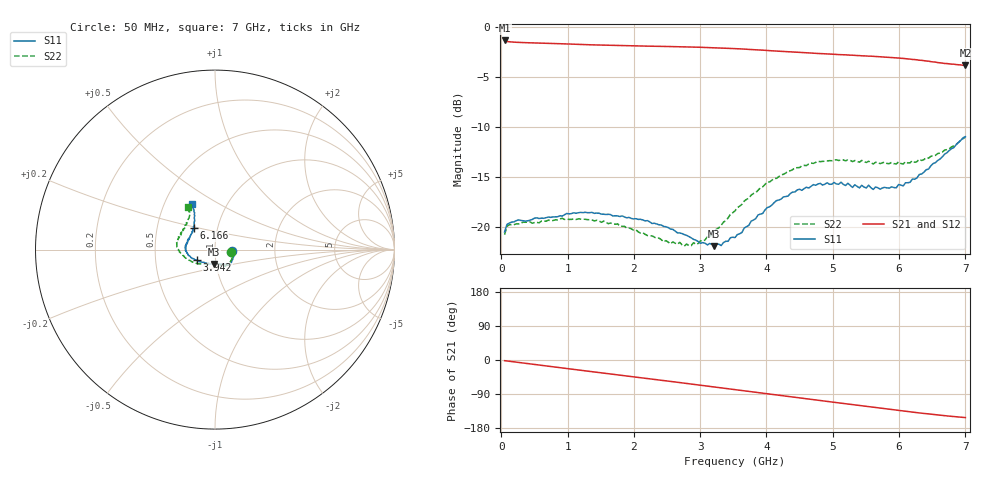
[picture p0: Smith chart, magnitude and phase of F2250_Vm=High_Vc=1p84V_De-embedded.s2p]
! Integrated Device Technology
! Corporate Headquarters
! 6024 Silver Creek Valley Road
! San Jose, CA 95138  USA
! Phone:  1-408-284-8200
! Toll Free:  1-800-223-1366
! Webpage:  http://www.idt.com/
! Timing and RF Division
! 515 Groton Road, Suite 102
! Westford, MA 01886-6024
! Device:  F2250
! Description: Voltage Variable RF Attenuator
! Frequency:  50.0 -  6000.00 MHz
! Package:  3x3 mm Thin QFN Plastic Package: 16 pin
! Ports:  2 RF, 3 DC
!  Pin  1  = GND
!  Pin  2  = NC
!  Pin  3  = RF1  = Port 1
!  Pin  4  = NC
!  Pin  5  = GND
!  Pin  6  = GND
!  Pin  7  = GND
!  Pin  8  = GND
!  Pin  9  = NC
!  Pin 10  = RF2  = Port 2
!  Pin 11  = NC
!  Pin 12  = GND
!  Pin 13  = GND
!  Pin 14  = VCNTRL
!  Pin 15  = VDD
!  Pin 16  = VMODE
! Vcntrl:  1.840 Volts
! Vmode:  +3.300 Volts
! Vdd:  +3.30  Volts
! Current:  1.324 mA
! Data:  The device was measured on a the F2250 evaluation board which has
!  individual transmission lines to the RF pins.  Data was collected
!  using a calibrated network analyzer.  The evaluation board was
!  de-embedded using a TRL calibration technique.
!  The reference plane is the edge of the package pin.
! Misc:  SN 10
!  Action Tracker AT0258
! Date Measured:  2014-11-26
! Date:  2015-10-15  MJV
! Note:
!  Integrated Device Technology supplies this data as a sample of measured
!  data at the package pin for this product.  Your particular data for this
!  product may vary.
!  Data was taken at 25 degrees C.
!  Integrated Device Technology reserves the right to change this data at anytime.
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# GHz S dB R 50
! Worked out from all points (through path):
!   201 points, 50 MHz to 7 GHz, reference 50 ohm
!   highest |S21| = -1.32 dB at 50 MHz (marker M1); lowest = -3.8 dB at 7 GHz (marker M2)
!   group delay of S21, straight-line fit = 61.1 ps
!   lowest |S11| = -21.9 dB at 3.212 GHz (marker M3), VSWR 1.17, Z = 48.8 - j7.88 ohm
!   |S11| at or under -10 dB: start of sweep to end of sweep
!   |S22| runs from -21.9 to -11.0 dB; largest |S21 - S12| = 0.0018
!   S11 on the Smith chart (normalised r, x): 50 MHz: 1.21, -0.02; 3.942 GHz: 0.81, -0.10; 6.166 GHz: 0.77, +0.19; 7 GHz: 0.69, +0.38
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0.05  -20.49 -5.8  -1.32 -1.8  -1.32 -1.8  -20.76 -7.0
0.08475  -19.73 -5.6  -1.42 -2.5  -1.42 -2.5  -19.93 -6.6
0.1195  -19.60 -6.3  -1.46 -3.3  -1.46 -3.3  -19.76 -6.6
0.71025  -18.99 -28.1  -1.61 -16.5  -1.61 -16.5  -19.30 -32.6
1.2315  -18.55 -43.1  -1.73 -27.9  -1.73 -27.9  -19.21 -52.2
1.75275  -18.88 -50.0  -1.83 -39.1  -1.83 -39.1  -19.67 -62.4
2.37825  -19.77 -52.9  -1.91 -52.6  -1.92 -52.6  -21.10 -72.0
2.552  -20.20 -56.4  -1.93 -56.5  -1.93 -56.5  -21.67 -78.4
2.86475  -21.08 -66.8  -1.98 -63.4  -1.98 -63.5  -21.85 -94.9
3.07325  -21.61 -80.8  -2.02 -68.2  -2.02 -68.2  -21.28 -110.1
3.21225  -21.91 -93.8  -2.05 -71.3  -2.05 -71.3  -20.42 -120.9
3.525  -21.05 -121.9  -2.14 -78.4  -2.14 -78.4  -18.37 -139.5
3.942  -18.64 -149.4  -2.29 -87.8  -2.30 -87.8  -15.98 -158.9
4.1505  -17.35 -158.4  -2.39 -92.4  -2.38 -92.5  -15.12 -167.2
4.4285  -16.48 -168.0  -2.49 -98.6  -2.49 -98.6  -14.07 -175.7
4.7065  -15.75 -176.4  -2.59 -104.7  -2.59 -104.7  -13.63 177.8
5.054  -15.68 175.1  -2.72 -112.4  -2.72 -112.4  -13.26 170.0
5.61  -16.23 158.1  -2.91 -124.5  -2.91 -124.6  -13.68 157.4
5.85325  -16.09 147.7  -3.01 -129.8  -3.02 -129.9  -13.65 150.3
6.166  -15.52 135.1  -3.19 -136.7  -3.19 -136.7  -13.56 141.5
6.54825  -13.55 123.5  -3.49 -144.5  -3.49 -144.6  -12.82 129.2
7  -10.95 117.0  -3.81 -151.9  -3.83 -152.0  -11.01 122.4
